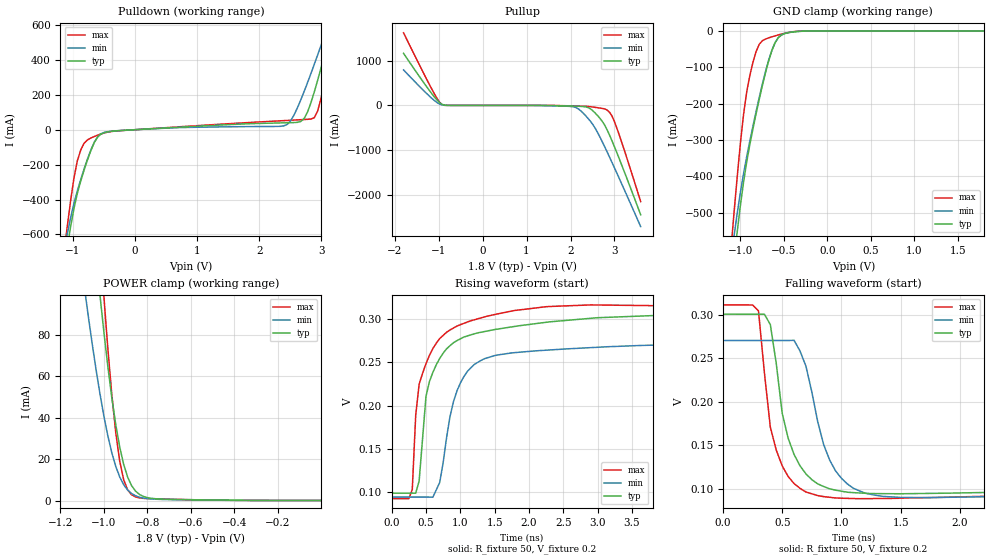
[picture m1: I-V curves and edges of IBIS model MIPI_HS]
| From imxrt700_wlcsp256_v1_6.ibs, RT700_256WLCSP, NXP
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[Model] MIPI_HS
Model_type   Output
Polarity   Non-Inverting
Enable   Active-High
Vmeas =   0.2
|Cref =   0
Rref =   50
|   typ   min   max
C_comp  6.36p   6.29p   6.40p
[Temperature Range]   85   125   -40
[Voltage Range]   1.8  1.52  1.98
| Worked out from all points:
|   slope of the pulldown table from 0 to 0.27 V, typ, clamps not added: 49.3 ohm
|   slope of the pullup table from 0 to 0.27 V, typ, clamps not added: 20.7 kohm
|   GND clamp passes 1 mA (typ) near -0.32 V on its own axis
|   POWER clamp passes 1 mA (typ) near -0.78 V on its own axis
|   falling waveform, R_fixture 50, V_fixture 0.2: 20-80 % time 169ps typ, 204ps min, 147ps max; typ from 0.301 V to 0.099 V
|   rising waveform, R_fixture 50, V_fixture 0.2: 20-80 % time 322ps typ, 328ps min, 296ps max; typ from 0.099 V to 0.301 V
[GND_clamp]
|Voltage   I (typ)   I (min)   I (max)
-1.8V     -2.465A    -2.105A    -2.739A
-1.109V   -713.7mA   -632.1mA   -604.8mA
-1.073V   -631.9mA   -565.4mA   -502mA
-1.036V   -554.2mA   -502.9mA   -403.4mA
-963.7mV  -417.6mA   -394mA     -231.6mA
-927.4mV  -361.8mA   -347.2mA   -169.1mA
-818.3mV  -227.5mA   -221.2mA   -56.37mA
-745.6mV  -149.4mA   -145.3mA   -26.52mA
-672.8mV  -81.15mA   -79.28mA   -18.73mA
-600.1mV  -32.11mA   -32.03mA   -13.25mA
-454.7mV  -4.969mA   -4.378mA   -4.395mA
1.8V      27.05uA    49.33uA    10.62uA
[Power_clamp]
|Volatge   I (typ)   I (min)   I (max)
-1.8V     1.169A     796.8mA    1.63A
-1.091V   181.3mA    104mA      247.2mA
-1.073V   159.7mA    89.82mA    215.5mA
-1.018V   99.42mA    51.6mA     125.7mA
-1V       81.35mA    40.79mA    98.51mA
-963.7mV  49.68mA    23.11mA    51.21mA
-945.5mV  36.65mA    16.49mA    32.78mA
-927.4mV  25.88mA    11.38mA    18.99mA
-891mV    11.36mA    5.082mA    5.159mA
-854.6mV  4.549mA    2.295mA    1.73mA
-745.6mV  748uA      559uA      757.1uA
-180uV    27.07uA    17.18uA    17.66uA
[Pulldown]
|Volatge   I (typ)   I (min)   I (max)
-1.8V     -2.466A    -2.106A    -2.74A
-1.091V   -675mA     -600.5mA   -557.9mA
-982.5mV  -451.6mA   -421.6mA   -276.6mA
-873.5mV  -294.1mA   -285.3mA   -116.5mA
-601mV    -41.86mA   -40.1mA    -31.35mA
2.397V    39.37mA    21.8mA     52.01mA
2.724V    63.99mA    218.7mA    58.42mA
2.887V    216.1mA    374.4mA    68.85mA
2.996V    354.3mA    482.7mA    180mA
3.105V    501.9mA    593mA      366.4mA
3.214V    654.1mA    704.6mA    570.8mA
3.595V    1.204A     1.102A     1.324A
[Pullup]
|Volatge   I (typ)   I (min)   I (max)
-1.8V     1.169A     797mA      1.63A
-1.146V   249.9mA    150.1mA    346.8mA
-928mV    26.48mA    11.7mA     19.82mA
1.797V    -8.515mA   -13.96mA   -5.212mA
2.179V    -18.78mA   -77.85mA   -14.35mA
2.397V    -46.78mA   -289.8mA   -22.77mA
2.56V     -170.4mA   -510.8mA   -43.36mA
2.778V    -444.6mA   -930.3mA   -77.8mA
2.887V    -665.5mA   -1.16A     -153.3mA
2.942V    -790.7mA   -1.276A    -234.8mA
3.159V    -1.327A    -1.751A    -813.6mA
3.595V    -2.454A    -2.72A     -2.158A
[Ramp]
|variable typ   min   max
dV/dt_r   120m/343p   106m/335p   132m/315p
dV/dt_f   123m/175p   109m/213p   132m/144p
R_load  = 50
[Falling waveform]
R_fixture = 50
V_fixture = 0.2
|time   V (typ)   V (min)   V (max)
0s        300.6mV    270.4mV    311.2mV
300ps     300.6mV    270.4mV    304.5mV
400ps     288.7mV    270.4mV    170.9mV
500ps     187mV      270.4mV    126.6mV
600ps     139.7mV    270.6mV    106.2mV
700ps     117.4mV    241.1mV    96.56mV
850ps     102.8mV    150.8mV    91.22mV
950ps     98.64mV    120.8mV    89.7mV
1.55ns    94.58mV    90.17mV    89.53mV
20ns      99.08mV    94.59mV    92.75mV
[Rising waveform]
R_fixture = 50
V_fixture = 0.2
|time   V (typ)   V (min)   V (max)
0s        99.1mV     94.59mV    92.73mV
300ps     99.1mV     94.58mV    103.3mV
350ps     99.1mV     94.58mV    188.7mV
400ps     113.1mV    94.58mV    224.8mV
500ps     210.8mV    94.58mV    248.3mV
650ps     247.1mV    103.1mV    271.9mV
900ps     272.4mV    204.4mV    289.4mV
1.05ns    278.9mV    233.2mV    294.7mV
1.8ns     291.4mV    261.1mV    309.7mV
20ns      300.5mV    270.4mV    311.3mV
